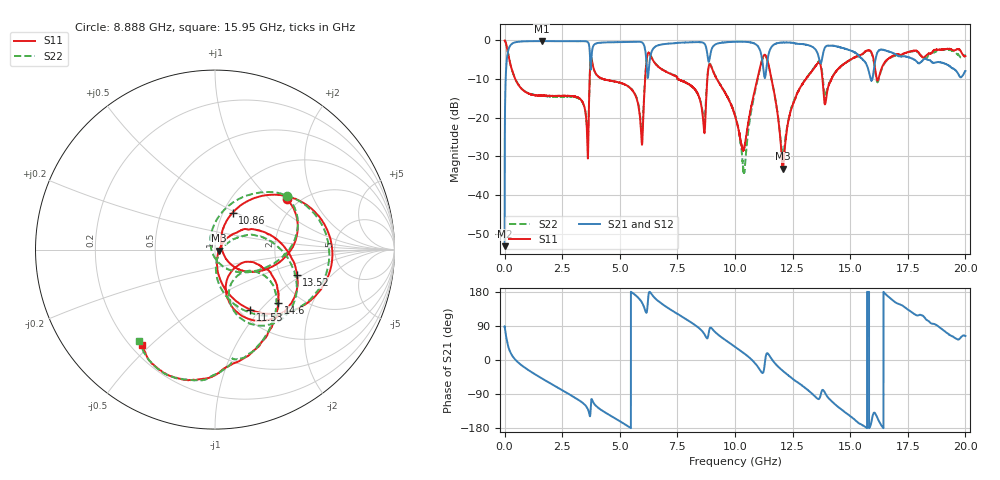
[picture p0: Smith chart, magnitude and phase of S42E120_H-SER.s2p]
!{S42E120}
!Johanson Technology Inc.
!www.johansontechnology.com
!Test Board Conditions:
!Substrate Type  RO4350B
!Substrate Thickness  50 mil
!Substrate Dk  3.66
!TL Type: GCPW
!TL Trace Width  60 mil
!TL Gap  10 mil
!Electrode orientation  Horizontal
!DUT TOPOLOGY	SERIES
!Mounting Pad LxW  14x55 mil
! Created Wed Nov 25 21:56:53 2020
# khz S ma R 50
! 2 Port Network Data from SP1.SP block
! freq  magS11  angS11  magS21  angS21  magS12  angS12  magS22  angS22
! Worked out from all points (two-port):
!   20001 points, 300 kHz to 20 GHz, reference 50 ohm
!   highest |S21| = -0.17 dB at 1.619 GHz (marker M1); lowest = -53.2 dB at 300 kHz (marker M2)
!   |S21| within 3 dB of the highest: 135.8 MHz to 3.698 GHz (3.562 GHz wide, 186 % of centre); 6.367 GHz to 8.789 GHz (2.422 GHz wide, 32 % of centre)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
!   lowest |S11| = -33.2 dB at 12.08 GHz (marker M3), VSWR 1.04, Z = 52.1 - j0.683 ohm
!   |S11| at or under -10 dB: 465.4 MHz to 3.692 GHz (3.227 GHz wide, 155 % of centre); 4.288 GHz to 6.098 GHz (1.811 GHz wide, 34.9 % of centre); 9.212 GHz to 10.97 GHz (1.758 GHz wide, 17.4 % of centre)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
!   |S22| runs from -34.3 to 0.0 dB; largest |S21 - S12| = 0.019
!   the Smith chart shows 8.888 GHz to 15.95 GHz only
!   S11 on the Smith chart (normalised r, x): 8.888 GHz: 1.72, +1.28; 10.86 GHz: 1.11, +0.48; 11.53 GHz: 1.12, -0.88; 13.52 GHz: 2.45, -0.89; 14.6 GHz: 1.55, -1.18; 15.95 GHz: 0.25, -0.47
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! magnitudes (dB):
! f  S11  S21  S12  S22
! 300 kHz  0.0  -53.2  -53.2  0.0
! 195.3 MHz  -4.7  -1.9  -1.9  -4.7
! 1.619 GHz  -14.3  -0.2  -0.2  -14.3
! 3.334 GHz  -15.5  -0.2  -0.2  -15.6
! 3.575 GHz  -23.4  -0.3  -0.3  -22.7
! 3.807 GHz  -5.8  -2.3  -2.3  -5.8
! 5.935 GHz  -24.8  -0.4  -0.4  -22.8
! 6.222 GHz  -3.3  -9.6  -9.7  -3.3
! 6.667 GHz  -6.8  -1.2  -1.3  -6.7
! 8.637 GHz  -21.9  -0.6  -0.7  -20.4
! 8.888 GHz  -6.2  -5.0  -5.0  -6.1
! 10 GHz  -19.4  -0.3  -0.3  -19.3
! 10.4 GHz  -27.8  -0.4  -0.4  -34.1
! 10.86 GHz  -12.8  -0.8  -0.8  -13.4
! 11.53 GHz  -8.2  -2.3  -2.3  -8.3
! 12.08 GHz  -33.2  -0.5  -0.5  -30.0
! 13.33 GHz  -8.0  -1.6  -1.6  -7.9
! 13.52 GHz  -6.4  -2.6  -2.6  -6.2
! 14.6 GHz  -6.7  -1.8  -1.8  -6.7
! 15.95 GHz  -3.5  -10.2  -10.1  -3.6
! 16.67 GHz  -4.7  -2.8  -3.0  -4.8
! 20 GHz  -4.1  -7.9  -7.8  -3.9
